FUNCTION_BLOCK FB_SDOWrite
VAR_IN_OUT 
	SDOWrite	:AccessSDO;		(* rising edge starts writing to the CoE Object *)
END_VAR
VAR_INPUT
	nSlaveAddr 	:UINT; 			(* Port Number of EtherCAT Slave *)
	sNetId     	:T_AmsNetId;	(* NetId of EtherCAT Master *)
END_VAR
VAR_OUTPUT
	bError		: BOOL;
    nErrId		: UDINT;
END_VAR
VAR
	fbSdoWrite 	:FB_EcCoESdoWrite;
END_VAR

fbSdoWrite(		sNetId:=sNetId,
				nSlaveAddr:=nSlaveAddr,
				nIndex:=SDOWrite.nIndex,
				nSubIndex  := SDOWrite.nSubIndex,
				pSrcBuf    := ADR(SDOWrite.nValue),
				cbBufLen   := SIZEOF(SDOWrite.nValue),
				bExecute   := SDOWrite.bExecute
		);

IF NOT fbSdoWrite.bBusy THEN
    SDOWrite.bExecute := FALSE;
    IF NOT fbSdoWrite.bError THEN 
        (* write successful *)
        bError := FALSE;
        nErrId := 0;
    ELSE 
        (* write failed *)
        bError := fbSdoWrite.bError;
        nErrId := fbSdoWrite.nErrId;
    END_IF
    fbSdoWrite(bExecute := FALSE);
END_IF

END_FUNCTION_BLOCK
